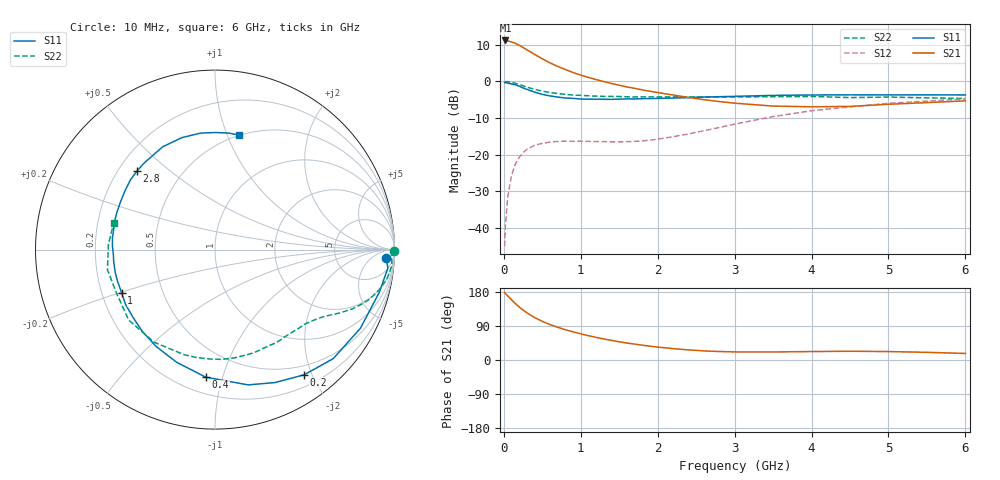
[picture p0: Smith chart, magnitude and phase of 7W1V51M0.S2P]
! Infineon Technologies  Discrete & RF Semiconductors
! BFS17W
! Si NPN RF Bipolar Junction Transistor in SOT323
! VCE = 1.5 V  IC = 1 mA
! Common Emitter S-Parameters:  August  1999
# GHz  S  MA  R  50
!  f  S11  S21  S12  S22
! GHz  MAG  ANG  MAG  ANG  MAG  ANG  MAG  ANG
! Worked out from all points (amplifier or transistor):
!   36 points, 10 MHz to 6 GHz, reference 50 ohm
!   highest |S21| = 11.2 dB at 20 MHz (marker M1)
!   |S21| within 3 dB of that: start of sweep to 335.9 MHz
!   unconditionally stable (mu >= 1): 983.4 MHz to end of sweep
!   at 250 MHz: K = 0.28, MSG = 14.4 dB, |S12| = -19.5 dB
!   at 1.4 GHz: K = 1.33, MAG = 4.5 dB, |S12| = -16.5 dB
!   at 6 GHz: K = 1.12, MAG = -2.4 dB, |S12| = -4.8 dB
!   S11 on the Smith chart (normalised r, x): 10 MHz: 20, -22; 200 MHz: 0.36, -1.89; 400 MHz: 0.31, -0.88; 1 GHz: 0.28, -0.20; 2.8 GHz: 0.28, +0.39; 6 GHz: 0.50, +1.10
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0.01  0.9552 -2.8  3.595 178.6  0.0056 87.7  0.9997 -0.5
0.02  0.9686 -6.1  3.617 175.7  0.0104 88.2  0.9834 -2.0
0.05  0.9461 -14.5  3.571 169.1  0.0264 82.1  0.99 -5.1
0.1  0.9212 -28.4  3.443 159.0  0.0519 73.4  0.9714 -9.9
0.15  0.896 -42.7  3.306 148.8  0.0741 65.3  0.9378 -14.2
0.2  0.8566 -54.5  3.111 139.8  0.0918 59.4  0.904 -17.8
0.25  0.8128 -65.7  2.898 131.8  0.1063 52.8  0.867 -20.8
0.3  0.7758 -76.3  2.698 124.5  0.118 48.3  0.8346 -23.3
0.4  0.7127 -94.1  2.333 112.0  0.1339 40.5  0.7769 -27.1
0.5  0.6632 -108.8  2.033 102.0  0.1422 35.2  0.7341 -29.9
0.6  0.6317 -121.2  1.786 93.5  0.148 31.6  0.7036 -32.4
0.8  0.5921 -140.8  1.449 79.9  0.1523 27.3  0.6635 -37.4
1  0.5732 -155.1  1.216 69.1  0.1521 26.2  0.643 -42.2
1.1  0.5709 -161.9  1.131 64.0  0.1512 26.5  0.6342 -45.2
1.6  0.5753 173.5  0.838 44.7  0.1497 33.1  0.6144 -60.1
2.2  0.5906 152.6  0.65 30.0  0.1752 47.4  0.6129 -79.7
2.8  0.6168 135.0  0.529 22.4  0.2342 54.8  0.6101 -100.1
3.5  0.6427 117.0  0.459 21.2  0.33 53.4  0.6176 -123.3
4  0.6506 106.5  0.449 22.3  0.3967 48.0  0.6209 -140.8
4.5  0.6541 96.9  0.454 23.1  0.4477 41.9  0.6 -156.3
5.5  0.6537 83.2  0.512 20.2  0.5378 30.0  0.5946 177.0
6  0.6514 78.0  0.541 17.3  0.573 24.4  0.5832 165.2
